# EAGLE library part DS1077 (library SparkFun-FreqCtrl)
I2C non-volatile programmable oscillator, 16kHz to 133MHz
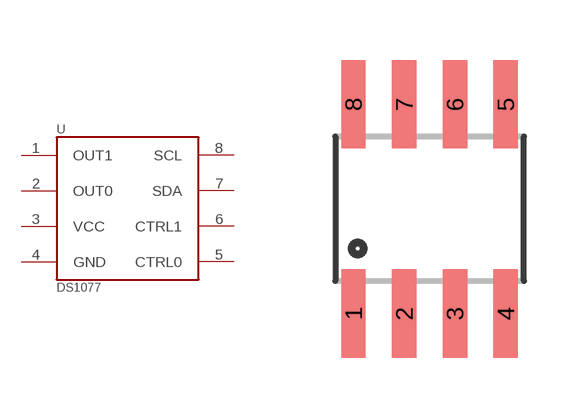
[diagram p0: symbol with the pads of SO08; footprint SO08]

Designator prefix -

## DS1077  [SO08]
1  OUT1
2  OUT0
3  VCC
4  GND
5  CTRL0
6  CTRL1
7  SDA
8  SCL

## Footprint SO08 (pad centres in mm)
Small Outline Package Fits JEDEC packages (narrow SOIC-8)
smd 0.61 x 2.21: 1 -1.905,-2.616; 2 -0.635,-2.616; 3 0.635,-2.616; 4 1.905,-2.616; 5 1.905,2.616; 6 0.635,2.616; 7 -0.635,2.616; 8 -1.905,2.616

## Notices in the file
Licensing: Creative Commons ShareAlike 4.0 International - https://creativecommons.org/licenses/by-sa/4.0
